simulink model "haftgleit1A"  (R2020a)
settings: Solver=ode45  StartTime=0.0  StopTime=4  RelTol=1e-6  AbsTol=1e-6
libraries: simulink x1

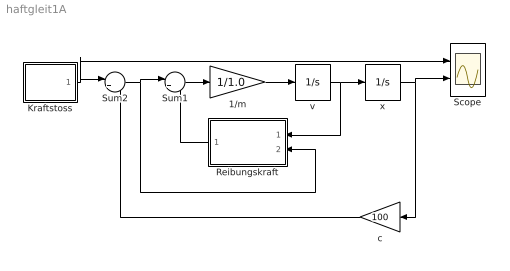
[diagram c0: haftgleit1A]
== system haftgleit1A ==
  1/m : Gain  Gain=1/1.0  SaturateOnIntegerOverflow=on
  Kraftstoss : Subsystem
  Reibungskraft : Subsystem
  Scope : Scope  NumInputPorts=2
  Sum1 : Sum  Inputs=|++  InputSameDT=on  SaturateOnIntegerOverflow=on
  Sum2 : Sum  Inputs=|+-  InputSameDT=on  SaturateOnIntegerOverflow=on
  c : Gain  Gain=100  SaturateOnIntegerOverflow=on
  v : Integrator
  x : Integrator  InitialCondition=3.5  UpperSaturationLimit=100  LowerSaturationLimit=-100
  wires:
  x/1 -> c/1, Scope/2
  Sum1/1 -> 1/m/1
  v/1 -> x/1, Reibungskraft/1(v)
  1/m/1 -> v/1
  Reibungskraft/1(FR) -> Sum1/2
  c/1 -> Sum2/2
  Kraftstoss/1(Fstoss) -> Sum2/1, Scope/1
  Sum2/1 -> Sum1/1, Reibungskraft/2(Fext)

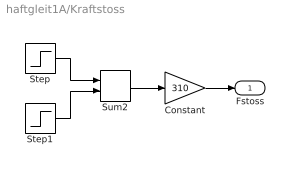
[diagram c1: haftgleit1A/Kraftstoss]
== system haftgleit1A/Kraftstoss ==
  Constant : Gain  Gain=310  SaturateOnIntegerOverflow=on
  Step : Step  Time=1.5  SampleTime=0
  Step1 : Step  Time=1.6  After=-1  SampleTime=0
  Sum2 : Sum  InputSameDT=on  SaturateOnIntegerOverflow=on
  Fstoss : Outport
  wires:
  Sum2/1 -> Constant/1
  Step/1 -> Sum2/1
  Step1/1 -> Sum2/2
  Constant/1 -> Fstoss/1

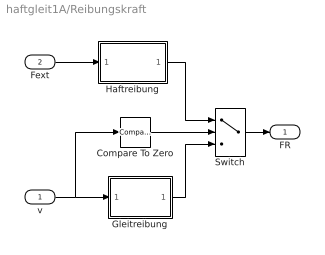
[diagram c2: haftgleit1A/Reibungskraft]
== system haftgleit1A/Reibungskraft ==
  v : Inport
  Fext : Inport  Port=2
  Compare To Zero : simulink/Logic and Bit Operations/Compare To Zero  relop===  OutDataTypeStr=uint8
  Gleitreibung : Subsystem
  Haftreibung : Subsystem
  Switch : Switch  Threshold=0.5
  FR : Outport
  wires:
  Switch/1 -> FR/1
  Fext/1 -> Haftreibung/1(Fext)
  v/1 -> Gleitreibung/1(v), Compare To Zero/1
  Haftreibung/1(Fh) -> Switch/1
  Gleitreibung/1(Fg) -> Switch/3
  Compare To Zero/1 -> Switch/2

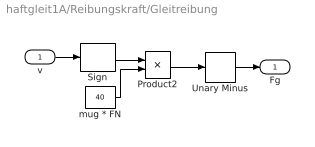
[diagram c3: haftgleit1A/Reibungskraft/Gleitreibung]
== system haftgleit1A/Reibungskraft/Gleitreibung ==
  v : Inport
  Product2 : Product  InputSameDT=on  SaturateOnIntegerOverflow=on
  Sign : Signum
  Unary Minus : UnaryMinus
  mug * FN : Constant  Value=40
  Fg : Outport
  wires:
  mug * FN/1 -> Product2/2
  Sign/1 -> Product2/1
  v/1 -> Sign/1
  Product2/1 -> Unary Minus/1
  Unary Minus/1 -> Fg/1

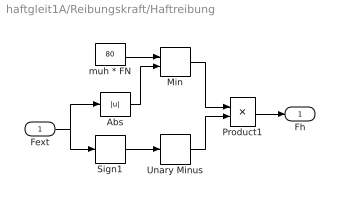
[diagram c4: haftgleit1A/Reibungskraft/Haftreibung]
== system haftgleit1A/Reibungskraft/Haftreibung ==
  Fext : Inport
  Abs : Abs
  Min : MinMax  Inputs=2  InputSameDT=on  SaturateOnIntegerOverflow=on
  Product1 : Product  InputSameDT=on  SaturateOnIntegerOverflow=on
  Sign1 : Signum
  Unary Minus : UnaryMinus
  muh * FN : Constant  Value=80
  Fh : Outport
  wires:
  Abs/1 -> Min/2
  muh * FN/1 -> Min/1
  Min/1 -> Product1/1
  Fext/1 -> Abs/1, Sign1/1
  Product1/1 -> Fh/1
  Sign1/1 -> Unary Minus/1
  Unary Minus/1 -> Product1/2
